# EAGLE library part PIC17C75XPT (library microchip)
MICROCONTROLLER
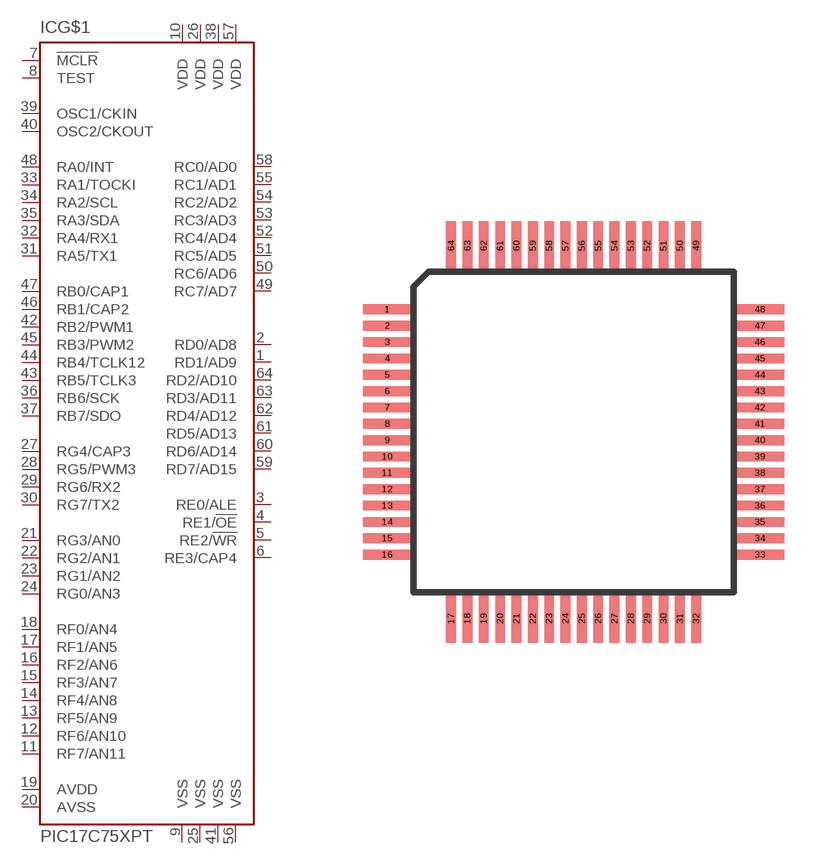
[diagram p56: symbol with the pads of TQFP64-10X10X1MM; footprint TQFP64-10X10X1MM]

Designator prefix IC; gates G$1=PIC17C75X P1=VDD P2=VDD P3=VDD P4=VDD P5=VSS P6=VSS P7=VSS P8=VSS

## PIC17C75XPTT (MF: MICROCHIP; MPN: PIC17C756A-33I/PT; OC_FARNELL: unknown; OC_NEWARK: 23C5980)  [TQFP64-10X10X1MM]
1  G$1:RD1/AD9
2  G$1:RD0/AD8
3  G$1:RE0/ALE
4  G$1:RE1/!OE
5  G$1:RE2/!WR
6  G$1:RE3/CAP4
7  G$1:!MCLR  in
8  G$1:TEST  in
9  P5:VSS  pwr
10  P1:VDD  pwr
11  G$1:RF7/AN11
12  G$1:RF6/AN10
13  G$1:RF5/AN9
14  G$1:RF4/AN8
15  G$1:RF3/AN7
16  G$1:RF2/AN6
17  G$1:RF1/AN5
18  G$1:RF0/AN4
19  G$1:AVDD  pwr
20  G$1:AVSS  pwr
21  G$1:RG3/AN0
22  G$1:RG2/AN1
23  G$1:RG1/AN2
24  G$1:RG0/AN3
25  P6:VSS  pwr
26  P2:VDD  pwr
27  G$1:RG4/CAP3
28  G$1:RG5/PWM3
29  G$1:RG6/RX2
30  G$1:RG7/TX2
31  G$1:RA5/TX1
32  G$1:RA4/RX1
33  G$1:RA1/TOCKI  in
34  G$1:RA2/SCL
35  G$1:RA3/SDA
36  G$1:RB6/SCK
37  G$1:RB7/SDO
38  P3:VDD  pwr
39  G$1:OSC1/CKIN  in
40  G$1:OSC2/CKOUT  out
41  P7:VSS  pwr
42  G$1:RB2/PWM1
43  G$1:RB5/TCLK3
44  G$1:RB4/TCLK12
45  G$1:RB3/PWM2
46  G$1:RB1/CAP2
47  G$1:RB0/CAP1
48  G$1:RA0/INT  in
49  G$1:RC7/AD7
50  G$1:RC6/AD6
51  G$1:RC5/AD5
52  G$1:RC4/AD4
53  G$1:RC3/AD3
54  G$1:RC2/AD2
55  G$1:RC1/AD1
56  P8:VSS  pwr
57  P4:VDD  pwr
58  G$1:RC0/AD0
59  G$1:RD7/AD15
60  G$1:RD6/AD14
61  G$1:RD5/AD13
62  G$1:RD4/AD12
63  G$1:RD3/AD11
64  G$1:RD2/AD10

## Footprint TQFP64-10X10X1MM (pad centres in mm)
64-Lead Plastic Thin Quad Flatpak (PT) - 10x10x1 mm Body Auto generated by make-symbol-device-package-bsdl.ulp Rev. 37 Source: http://ww1.microchip.com/downloads/en/DeviceDoc/61143G.pdf
smd 1.5 x 0.3: 1 -5.7,3.75; 2 -5.7,3.25; 3 -5.7,2.75; 4 -5.7,2.25; 5 -5.7,1.75; 6 -5.7,1.25; 7 -5.7,0.75; 8 -5.7,0.25; 9 -5.7,-0.25; 10 -5.7,-0.75; 11 -5.7,-1.25; 12 -5.7,-1.75; 13 -5.7,-2.25; 14 -5.7,-2.75; 15 -5.7,-3.25; 16 -5.7,-3.75; 33 5.7,-3.75; 34 5.7,-3.25; 35 5.7,-2.75; 36 5.7,-2.25; 37 5.7,-1.75; 38 5.7,-1.25; 39 5.7,-0.75; 40 5.7,-0.25; 41 5.7,0.25; 42 5.7,0.75; 43 5.7,1.25; 44 5.7,1.75; 45 5.7,2.25; 46 5.7,2.75; 47 5.7,3.25; 48 5.7,3.75
smd 0.3 x 1.5: 17 -3.75,-5.7; 18 -3.25,-5.7; 19 -2.75,-5.7; 20 -2.25,-5.7; 21 -1.75,-5.7; 22 -1.25,-5.7; 23 -0.75,-5.7; 24 -0.25,-5.7; 25 0.25,-5.7; 26 0.75,-5.7; 27 1.25,-5.7; 28 1.75,-5.7; 29 2.25,-5.7; 30 2.75,-5.7; 31 3.25,-5.7; 32 3.75,-5.7; 49 3.75,5.7; 50 3.25,5.7; 51 2.75,5.7; 52 2.25,5.7; 53 1.75,5.7; 54 1.25,5.7; 55 0.75,5.7; 56 0.25,5.7; 57 -0.25,5.7; 58 -0.75,5.7; 59 -1.25,5.7; 60 -1.75,5.7; 61 -2.25,5.7; 62 -2.75,5.7; 63 -3.25,5.7; 64 -3.75,5.7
